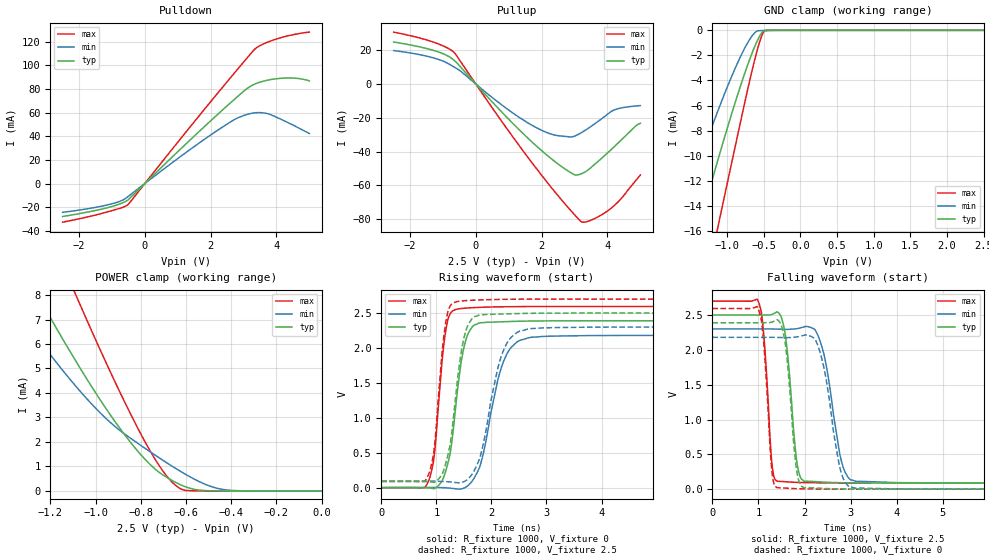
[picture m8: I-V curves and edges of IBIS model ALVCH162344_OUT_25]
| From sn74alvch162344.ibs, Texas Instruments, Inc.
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[Model]   ALVCH162344_OUT_25
Model_type  3-state
Enable   Active-Low
Vref =   0
Rref =   500
Cref =   30
Vmeas =   1.25
| variable   typ   min   max
C_comp   3.68pF   3.18pF   3.96pF
| C_pullup   1.58pF   0.97pF   2.96pF
| C_pulldown   0.86pF   0.70pF   1.15pF
| C_tri-state   3.68pF   3.18pF   3.96pF
[Temperature Range]   40   100   -40
| Ambient temperature   25   85   -40
[Voltage range]   2.5   2.3   2.7
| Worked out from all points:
|   slope of the pulldown table from 0 to 0.375 V, typ, clamps not added: 36.9 ohm
|   slope of the pullup table from 0 to 0.375 V, typ, clamps not added: 46.7 ohm
|   GND clamp passes 1 mA (typ) near -0.60 V on its own axis
|   POWER clamp passes 1 mA (typ) near -0.75 V on its own axis
|   rising waveform, R_fixture 1000, V_fixture 0: 20-80 % time 229ps typ, 355ps min, 170ps max; typ from 0 V to 2.39 V
|   falling waveform, R_fixture 1000, V_fixture 2.5: 20-80 % time 182ps typ, 311ps min, 143ps max; typ from 2.5 V to 0.089 V
|   rising waveform, R_fixture 1000, V_fixture 2.5: 20-80 % time 231ps typ, 346ps min, 169ps max; typ from 0.089 V to 2.5 V
|   falling waveform, R_fixture 1000, V_fixture 0: 20-80 % time 178ps typ, 308ps min, 143ps max; typ from 2.39 V to 0 V
[GND Clamp]
| ALVCH162344_OUT_25
|   Voltage   I(typ)   I(min)   I(max)
-2.5V     -40.61mA   -30.07mA   -55.51mA
-1.69V    -22.33mA   -15.67mA   -31.65mA
-1.65V    -21.45mA   -14.99mA   -30.5mA
-1.37V    -15.42mA   -10.3mA    -22.53mA
-1.13V    -10.45mA   -6.501mA   -15.84mA
-1.1V     -9.846mA   -6.045mA   -15.02mA
-795mV    -4.057mA   -1.838mA   -6.74mA
-680mV    -2.145mA   -624.5uA   -3.733mA
-595mV    -929.2uA   -73.58uA   -1.727mA
-525mV    -184.8uA   -21.15uA   -417uA
-480mV    -14.4uA    -14.03uA   -14.71uA
2.5V      81.29pA    49.99nA    36.69pA
[POWER Clamp]
| ALVCH162344_OUT_25
|   Voltage   I(typ)   I(min)   I(max)
-2.5V     31.6mA     24.86mA    42.33mA
-1.39V    10.28mA    7.981mA    14.75mA
-1.265V   8.15mA     6.364mA    11.9mA
-1.24V    7.735mA    6.053mA    11.34mA
-1.09V    5.346mA    4.307mA    8.068mA
-950mV    3.315mA    2.929mA    5.172mA
-825mV    1.754mA    2.021mA    2.776mA
-720mV    769.6uA    1.36mA     1.055mA
-640mV    322.9uA    888.6uA    184.5uA
-555mV    52.44uA    443.5uA    3.317uA
-425mV    558.3nA    44.67uA    18.75nA
-31.15fV  81.29pA    293.6pA    44pA
[Pulldown]
| ALVCH162344_OUT_25
|   Voltage   I(typ)   I(min)   I(max)
-2.5V     -27.91mA   -24.39mA   -32.71mA
-1.095V   -20.15mA   -17.8mA    -23.69mA
-715mV    -16.8mA    -14.53mA   -20.55mA
-505mV    -13.71mA   -10.91mA   -17.61mA
830mV     22.38mA    17.61mA    29.02mA
1.89V     50.21mA    38.94mA    65.48mA
2.71V     70.9mA     53.9mA     93.07mA
3.075V    79.69mA    58.13mA    105.1mA
3.36V     84.37mA    59.87mA    114.1mA
3.66V     86.97mA    59.53mA    118.8mA
4.39V     89.29mA    51mA       125.2mA
5V        86.82mA    42.29mA    128.1mA
[Pullup]
| ALVCH162344_OUT_25
|   Voltage   I(typ)   I(min)   I(max)
-2.5V     24.97mA    19.88mA    30.85mA
-1.26V    19.83mA    15.39mA    24.7mA
-660mV    14.06mA    10.13mA    18.67mA
920mV     -19.27mA   -14.27mA   -25.76mA
1.86V     -37.05mA   -26.04mA   -50.56mA
2.54V     -47.97mA   -30.69mA   -67.15mA
2.995V    -53.7mA    -30.84mA   -77.37mA
3.2V      -53.21mA   -28.86mA   -81.55mA
3.535V    -48.83mA   -24.61mA   -80.36mA
4.09V     -39.2mA    -16.54mA   -73.89mA
4.42V     -33.1mA    -14.12mA   -67.8mA
5V        -23.23mA   -12.73mA   -53.86mA
[Ramp]
| ALVCH162344_OUT_25
| variable   typ   min   max
dV/dt_r   1.44/2.37E-10   1.32/3.81E-10   1.56/1.79E-10
dV/dt_f   1.47/1.94E-10   1.35/3.22E-10   1.58/1.54E-10
R_load = 1000
[Rising Waveform]
| ALVCH162344_OUT_25
R_fixture =   1000
C_fixture =   0
L_fixture =   0
V_fixture =   0
V_fixture_min = 0
V_fixture_max = 0
|   Time   V(typ)   V(min)   V(max)
0s        246.9nV    5.631uV    -61.89nV
850ps     -3.855mV   1.958mV    80.92mV
955ps     -13.83mV   3.24mV     415.3mV
1.185ns   278.5mV    -3.641mV   2.315V
1.435ns   1.712V     -20.82mV   2.563V
1.57ns    2.193V     26.23mV    2.573V
1.785ns   2.358V     291.8mV    2.581V
2.265ns   2.377V     1.888V     2.59V
2.735ns   2.386V     2.154V     2.593V
24.99ns   2.39V      2.18V      2.594V
[Falling Waveform]
| ALVCH162344_OUT_25
R_fixture =   1000
C_fixture =   0
L_fixture =   0
V_fixture =   2.5
V_fixture_min = 2.3
V_fixture_max = 2.7
|   Time   V(typ)   V(min)   V(max)
0s        2.5V       2.3V       2.7V
1.005ns   2.499V     2.3V       2.682V
1.295ns   2.509V     2.3V       353.5mV
1.415ns   2.542V     2.298V     113mV
1.84ns    359mV      2.305V     97.08mV
2.005ns   112.3mV    2.334V     94.14mV
2.35ns    103.1mV    2.102V     91.29mV
2.8ns     92.44mV    404mV      90.05mV
3.115ns   90.05mV    111.9mV    89.78mV
24.99ns   88.67mV    89.46mV    89.88mV
[Rising Waveform]
| ALVCH162344_OUT_25
R_fixture =   1000
C_fixture =   0
L_fixture =   0
V_fixture =   2.5
V_fixture_min = 2.3
V_fixture_max = 2.7
|   Time   V(typ)   V(min)   V(max)
0s        88.62mV    89.39mV    89.85mV
850ps     84.61mV    91.01mV    172.8mV
955ps     75.3mV     92.05mV    518.2mV
1.18ns    373.1mV    85.52mV    2.409V
1.43ns    1.828V     69.5mV     2.67V
1.57ns    2.321V     121mV      2.679V
1.785ns   2.472V     415.3mV    2.688V
2.235ns   2.487V     1.994V     2.696V
2.71ns    2.496V     2.277V     2.699V
24.99ns   2.5V       2.3V       2.7V
[Falling Waveform]
| ALVCH162344_OUT_25
R_fixture =   1000
C_fixture =   0
L_fixture =   0
V_fixture =   0
V_fixture_min = 0
V_fixture_max = 0
|   Time   V(typ)   V(min)   V(max)
0s        2.39V      2.18V      2.594V
1ns       2.389V     2.18V      2.582V
1.295ns   2.398V     2.18V      241.5mV
1.415ns   2.43V      2.178V     20.06mV
1.59ns    2.052V     2.175V     15.14mV
1.835ns   245.5mV    2.186V     6.576mV
2ns       18.23mV    2.211V     3.878mV
2.31ns    14.01mV    2.023V     1.423mV
3.1ns     1.1mV      13.26mV    -100.3uV
24.99ns   280.6nV    324.9nV    216.7nV
